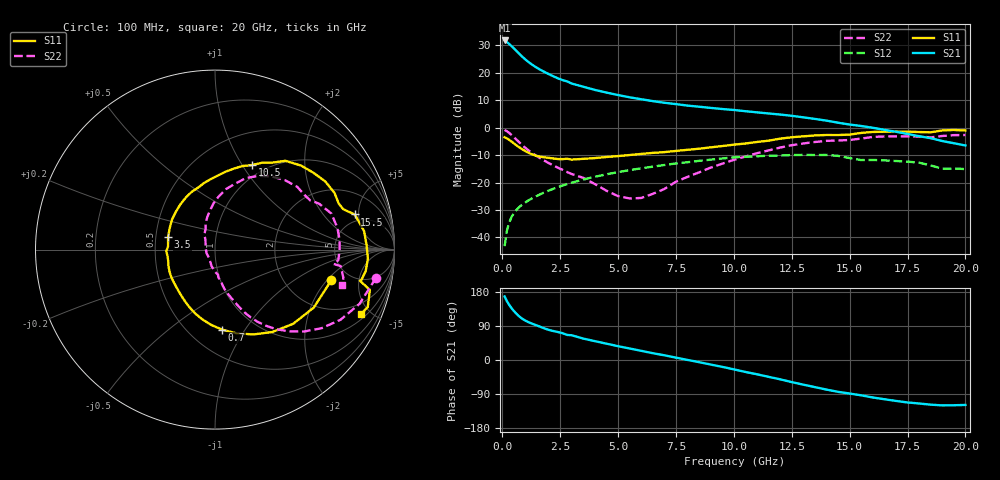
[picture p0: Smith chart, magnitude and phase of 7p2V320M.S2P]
! Infineon Technologies  Discrete & RF Semiconductors
! bfp620
! VCE =  2.3 V,  IC =  20 mA
! Common Emitter S-Parameters:  Sep 2002
# GHz  S  MA  R  50
!  f  S11  S21  S12  S22
! GHz  MAG  ANG  MAG  ANG  MAG  ANG  MAG  ANG
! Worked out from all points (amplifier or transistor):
!   59 points, 100 MHz to 20 GHz, reference 50 ohm
!   highest |S21| = 31.8 dB at 100 MHz (marker M1)
!   |S21| within 3 dB of that: start of sweep to 511.5 MHz
!   unconditionally stable (mu >= 1): 3.011 GHz to 10.01 GHz; 17.16 GHz to end of sweep
!   at 1 GHz: K = 0.70, MSG = 26.1 dB, |S12| = -27.2 dB
!   at 5.5 GHz: K = 1.04, MAG = 12.0 dB, |S12| = -15.5 dB
!   at 20 GHz: K = 1.27, MAG = 1.2 dB, |S12| = -15.1 dB
!   S11 on the Smith chart (normalised r, x): 100 MHz: 3.61, -2.23; 700 MHz: 0.71, -0.80; 3.5 GHz: 0.58, +0.09; 10.5 GHz: 0.87, +1.11; 15.5 GHz: 4.07, +4.48; 20 GHz: 1.28, -4.39
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0.1  0.6705 -14.7  39.08 167.6  0.0069 60.6  0.9112 -9.9
0.2  0.6382 -30.4  36.45 155.3  0.0133 65.2  0.8599 -20.6
0.3  0.6005 -43.5  33.67 145.3  0.0187 64.4  0.8012 -29.2
0.4  0.5592 -55.2  30.8 136.8  0.0235 62.7  0.7379 -36.4
0.5  0.5184 -65.8  27.98 129.3  0.0276 61.1  0.6743 -42.6
0.6  0.481 -75.7  25.36 122.7  0.0313 59.6  0.6138 -47.9
0.7  0.4482 -84.8  22.99 116.8  0.0346 58.4  0.5585 -52.5
0.8  0.4197 -93.0  20.91 111.7  0.0378 57.5  0.5092 -56.3
1  0.3734 -106.9  17.54 103.8  0.0435 56.1  0.4287 -62.1
1.2  0.3384 -118.2  15.03 98.0  0.049 55.3  0.3682 -65.9
1.6  0.2982 -137.3  11.69 88.6  0.06 53.9  0.2841 -71.4
2  0.2823 -153.6  9.551 79.6  0.0711 52.1  0.2269 -76.4
2.4  0.2682 -166.7  7.971 73.9  0.0823 49.9  0.1868 -78.9
2.8  0.2716 -177.9  6.983 66.2  0.0938 47.4  0.1554 -83.4
3.5  0.2705 165.0  5.584 56.4  0.1136 42.2  0.1217 -90.5
5  0.3037 135.6  3.941 36.4  0.1549 29.7  0.0565 -127.0
7  0.3587 104.9  2.854 12.4  0.2086 11.8  0.0762 134.4
10.5  0.5149 66.2  2.001 -31.6  0.2953 -26.3  0.2982 85.8
13.5  0.7222 31.7  1.448 -71.5  0.3187 -61.8  0.5488 44.9
15.5  0.8029 14.1  1.075 -93.2  0.2568 -83.6  0.6334 23.9
17  0.8534 -3.4  0.844 -108.0  0.247 -93.5  0.6962 4.7
20  0.8894 -23.8  0.474 -118.6  0.1762 -103.6  0.7365 -15.5
